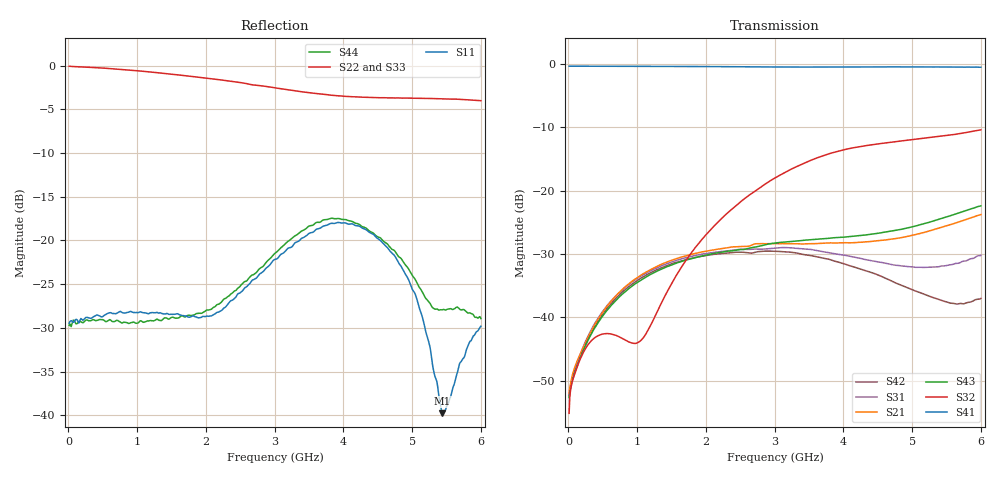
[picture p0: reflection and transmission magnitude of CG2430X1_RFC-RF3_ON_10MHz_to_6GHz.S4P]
!CEL
!CG2430X1
!Port1: RFC Port2: RF1  Port3: RF2 Port4: RF3
!Data & Calibration Information:
!Freq	S11:SOLT4(ON)	S12:SOLT4(ON)	S13:SOLT4(ON)	S14:SOLT4(ON)
!	S21:SOLT4(ON)	S22:SOLT4(ON)	S23:SOLT4(ON)	S24:SOLT4(ON)
!	S31:SOLT4(ON)	S32:SOLT4(ON)	S33:SOLT4(ON)	S34:SOLT4(ON)
!	S41:SOLT4(ON)	S42:SOLT4(ON)	S43:SOLT4(ON)	S44:SOLT4(ON)
# Hz S dB R 50
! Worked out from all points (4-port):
!   600 points, 10 MHz to 6 GHz, reference 50 ohm
!   strongest paths, dB at 10 MHz, 1.51 GHz, 3.01 GHz, 4.51 GHz, 6 GHz:
!     S41: -0.4, -0.4, -0.5, -0.5, -0.5
!     S32: -55.2, -34.5, -18.0, -12.6, -10.4
!     S43: -52.7, -31.7, -28.3, -26.7, -22.4
!     S21: -52.0, -31.0, -28.4, -27.9, -23.8
!     S31: -52.3, -31.2, -29.1, -31.3, -30.2
!     S42: -52.4, -31.5, -29.6, -33.4, -37.0
!   lowest |S11| = -39.8 dB at 5.44 GHz (marker M1), VSWR 1.02, Z = 50.8 - j0.599 ohm
!   |S11| at or under -10 dB: start of sweep to end of sweep
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1e7  -29.47 -0.0  -52.09 13.6  -52.29 11.9  -0.39 -0.4
     -52.00 14.5  -0.08 -0.6  -55.28 51.4  -52.48 14.3
     -52.27 12.6  -55.18 50.1  -0.07 -0.6  -52.72 12.8
     -0.37 -0.2  -52.42 14.0  -52.69 12.5  -29.73 -3.3
6.4e8  -28.36 16.5  -37.22 66.4  -37.20 54.4  -0.39 -5.5
       -37.24 66.7  -0.37 -27.2  -42.70 3.8  -37.64 55.2
       -37.21 54.4  -42.71 3.8  -0.35 -26.8  -37.98 66.4
       -0.38 -5.6  -37.62 55.2  -37.94 66.1  -29.28 21.5
1.87e9  -28.80 8.5  -29.91 56.4  -30.21 22.2  -0.42 -15.4
        -29.87 56.2  -1.32 -76.2  -28.66 -169.2  -30.53 24.0
        -30.21 22.1  -28.68 -169.2  -1.29 -75.9  -30.51 59.7
        -0.42 -15.4  -30.52 23.5  -30.53 59.9  -28.35 12.4
4.13e9  -18.11 43.4  -28.30 56.6  -30.44 -57.1  -0.50 -33.6
        -28.24 56.8  -3.58 -162.3  -13.29 103.0  -31.97 -49.4
        -30.46 -57.1  -13.28 102.9  -3.58 -162.1  -27.20 59.2
        -0.51 -33.7  -31.99 -49.5  -27.22 58.8  -17.83 45.3
4.94e9  -24.36 36.1  -27.15 68.5  -32.04 -92.5  -0.46 -40.9
        -27.21 68.5  -3.73 172.7  -12.05 81.8  -35.36 -80.8
        -32.01 -92.4  -12.04 81.7  -3.66 174.3  -25.94 65.7
        -0.47 -41.0  -35.39 -81.6  -25.88 65.5  -23.15 18.7
5.44e9  -39.77 -35.0  -25.68 73.9  -31.92 -116.2  -0.49 -45.9
        -25.77 74.1  -3.82 161.9  -11.39 72.0  -37.41 -108.4
        -31.91 -115.4  -11.40 72.1  -3.79 164.6  -24.48 68.5
        -0.50 -46.0  -37.41 -108.2  -24.38 68.4  -27.94 -41.2
6e9  -29.81 -143.7  -23.79 76.4  -30.22 -141.2  -0.53 -51.4
     -23.80 76.4  -4.02 151.6  -10.45 61.7  -37.21 -144.3
     -30.24 -141.1  -10.42 61.3  -4.13 154.1  -22.41 67.0
     -0.53 -51.5  -37.04 -145.4  -22.42 67.9  -28.93 -91.2
